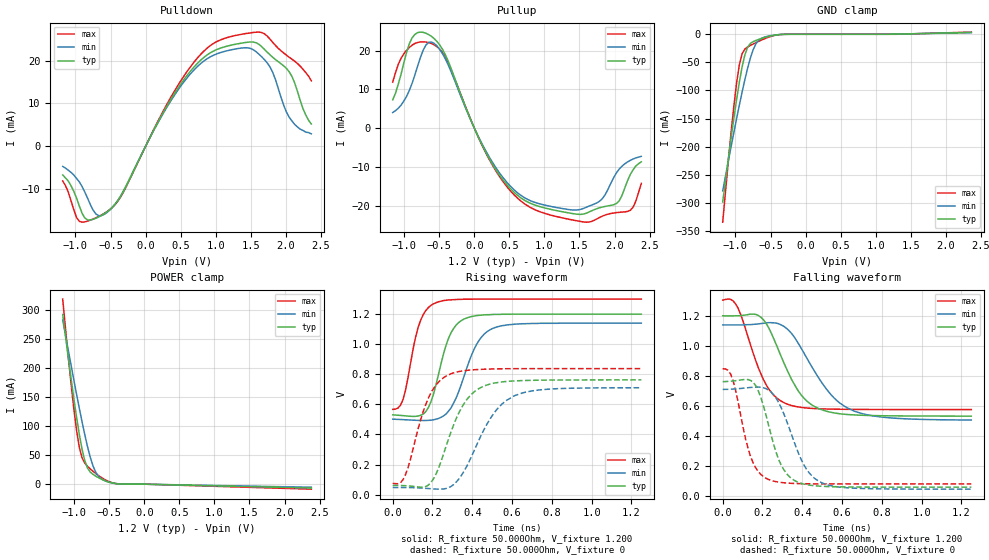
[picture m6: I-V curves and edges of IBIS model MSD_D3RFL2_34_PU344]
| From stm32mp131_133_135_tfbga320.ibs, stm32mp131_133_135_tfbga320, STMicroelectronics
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[Model] MSD_D3RFL2_34_PU344
Model_type   I/O
C_comp 2.348pF   2.261pF   2.473pF
Vinh = 820.000mV
Vinl = 380.000mV
Vmeas = 600.000mV
Vref = 600.000mV
[Model Spec]
Vinh   820.000mV   790.000mV   870.000mV
Vinl   380.000mV   350.000mV   430.000mV
Vmeas   600.000mV   570.000mV   650.000mV
Vref   600.000mV   570.000mV   650.000mV
[Receiver Thresholds]
Vth   =  0.600V
Vth_min  =  0.5880V
Vth_max  =  0.6120V
Vinh_ac  =  0.220V
Vinh_dc  =  0.130V
Vinl_ac  = -0.220V
Vinl_dc  = -0.130V
Tslew_ac =  5.000ns |Not specified, so set to high value
[Temperature Range]   25.000   125.000   -40.000
[Voltage Range]   1.200V   1.140V   1.300V
[GND Clamp Reference]   0.00V   0.00V   0.00V
[Pulldown Reference]   0.00V   0.00V   0.00V
[POWER Clamp Reference]   1.200V   1.140V   1.300V
[Pullup Reference]   1.200V   1.140V   1.300V
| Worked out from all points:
|   slope of the pulldown table from 0 to 0.18 V, typ, clamps not added: 31.3 ohm
|   slope of the pullup table from 0 to 0.18 V, typ, clamps not added: 26.5 ohm
|   GND clamp passes 1 mA (typ) near -0.41 V on its own axis
|   POWER clamp passes 1 mA (typ) near -0.41 V on its own axis
|   rising waveform, R_fixture 50.000Ohm, V_fixture 1.200: 20-80 % time 85.8ps typ, 114ps min, 71.8ps max; typ from 0.53 V to 1.2 V
|   rising waveform, R_fixture 50.000Ohm, V_fixture 0: 20-80 % time 130ps typ, 163ps min, 109ps max; typ from 0.061 V to 0.763 V
|   falling waveform, R_fixture 50.000Ohm, V_fixture 1.200: 20-80 % time 149ps typ, 195ps min, 124ps max; typ from 1.2 V to 0.533 V
|   falling waveform, R_fixture 50.000Ohm, V_fixture 0: 20-80 % time 96.8ps typ, 124ps min, 82.6ps max; typ from 0.762 V to 0.06 V
[GND Clamp]
-1.182V   -298.5mA   -278.7mA   -334.6mA
-1.064V   -186.4mA   -201mA     -176.4mA
-984.9mV  -117.1mA   -150.9mA   -87.65mA
-945.5mV  -85.8mA    -126.7mA   -54.89mA
-906.1mV  -58.45mA   -103.4mA   -34.82mA
-866.7mV  -36.99mA   -81.15mA   -26.46mA
-787.9mV  -16.43mA   -42.51mA   -19.96mA
-709.1mV  -11.02mA   -17.14mA   -14.94mA
-630.3mV  -7.563mA   -7.255mA   -10.33mA
-512.1mV  -3.391mA   -2.874mA   -4.513mA
-315.1mV  -135.6uA   -195uA     -130uA
2.364V    3.306mA    2.793mA    3.888mA
[Power Clamp]
-1.164V   291.7mA    282.1mA    318.2mA
-1.085V   217.9mA    230.5mA    219.1mA
-1.006V   147.8mA    179.6mA    130.3mA
-966.7mV  115.4mA    154.8mA    92.58mA
-927.3mV  85.61mA    130.5mA    63.27mA
-887.9mV  59.92mA    107mA      45.21mA
-809.1mV  27.42mA    64.02mA    30.59mA
-730.3mV  16.72mA    30.92mA    21.98mA
-690.9mV  13.66mA    20.11mA    18.17mA
-572.7mV  6.48mA     6.432mA    8.549mA
-336.4mV  188.5uA    360.2uA    208.2uA
2.382V    -6.618mA   -5.26mA    -8.576mA
[Pulldown]
-1.182V   -6.7mA     -4.7mA     -8.1mA
-945.5mV  -13.93mA   -8.3mA     -17.52mA
-866.7mV  -16.74mA   -10.69mA   -17.66mA
-709.1mV  -16.81mA   -15.8mA    -16.7mA
-551.5mV  -15.32mA   -15.48mA   -15.28mA
-354.6mV  -11.64mA   -11.56mA   -11.82mA
551.5mV   15.66mA    15.14mA    16.51mA
906.1mV   21.64mA    20.72mA    23.3mA
1.261V    23.76mA    22.65mA    25.79mA
1.733V    22.01mA    19.52mA    25.76mA
2.009V    18.18mA    7.99mA     21.28mA
2.364V    5.2mA      2.9mA      15.3mA
[Pullup]
-1.164V   7.3mA      4.009mA    11.85mA
-887.9mV  23.27mA    11.54mA    21.41mA
-730.3mV  24.71mA    20.07mA    22.27mA
-612.1mV  23.69mA    22.22mA    21.84mA
-375.8mV  17.41mA    16.45mA    16.97mA
215.2mV   -7.946mA   -7.528mA   -8.167mA
727.3mV   -18.75mA   -18.09mA   -19.68mA
1.515V    -22.28mA   -20.98mA   -24.1mA
1.791V    -20.54mA   -18.82mA   -23.03mA
1.988V    -19.79mA   -12.79mA   -21.91mA
2.224V    -12mA      -8.343mA   -21.22mA
2.382V    -8.7mA     -7.295mA   -14.29mA
[Ramp]
R_load=50.000Ohm
dV/dt_r   410.958mV/108.000ps  389.622mV/139.000ps  443.955mV/90.500ps
dV/dt_f   410.958mV/123.500ps  389.559mV/161.000ps  443.955mV/103.500ps
[Rising waveform]
R_fixture=50.000Ohm
V_fixture=1.200
V_fixture_min=1.140
V_fixture_max=1.300
0s        530.1mV    501.7mV    566.7mV
52ps      525.1mV    498.5mV    632.8mV
115ps     520.5mV    494.3mV    1.047V
154ps     536mV      492.7mV    1.198V
218ps     731.7mV    501.6mV    1.276V
269ps     996.8mV    537.4mV    1.292V
320ps     1.129V     645.7mV    1.297V
422ps     1.19V      999.5mV    1.3V
498ps     1.197V     1.102V     1.3V
1.25ns    1.2V       1.14V      1.3V
[Rising waveform]
R_fixture=50.000Ohm
V_fixture=0
0s        60.99mV    47.45mV    75.82mV
64ps      59.44mV    47.1mV     132.2mV
179ps     63.35mV    40.53mV    640.8mV
218ps     137.3mV    37.09mV    729.4mV
281ps     371.8mV    46.65mV    796.2mV
345ps     574.9mV    126.8mV    821.1mV
409ps     682.9mV    291.4mV    830.2mV
511ps     741.8mV    544.6mV    835.7mV
613ps     756mV      658mV      837.2mV
1.25ns    762.7mV    710.6mV    837.7mV
[Falling waveform]
R_fixture=50.000Ohm
V_fixture=1.200
V_fixture_min=1.140
V_fixture_max=1.300
0s        1.2V       1.139V     1.304V
77ps      1.2V       1.139V     1.251V
192ps     1.19V      1.148V     813.4mV
256ps     1.049V     1.153V     672mV
320ps     850mV      1.117V     614.8mV
435ps     620.1mV    890.4mV    585.1mV
537ps     560.2mV    686.9mV    579.5mV
626ps     543.4mV    588mV      577.9mV
805ps     535.1mV    525.5mV    576.5mV
1.25ns    532.6mV    506.7mV    576.3mV
[Falling waveform]
R_fixture=50.000Ohm
V_fixture=0
0s        762.1mV    710.2mV    847mV
52ps      766.2mV    712.5mV    769.3mV
115ps     776.6mV    719.9mV    381mV
154ps     755.9mV    724.9mV    218.5mV
230ps     475.5mV    706.4mV    111.6mV
281ps     245.1mV    623.7mV    93.84mV
320ps     152.6mV    505mV      87.96mV
409ps     80.46mV    206.5mV    83.09mV
498ps     66.14mV    89.7mV     81.97mV
1.25ns    60.35mV    46.92mV    81.65mV
